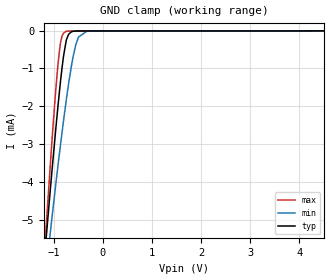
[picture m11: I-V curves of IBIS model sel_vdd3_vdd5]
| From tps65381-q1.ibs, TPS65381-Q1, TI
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|   sel_vdd3_vdd5 Model
[Model]   sel_vdd3_vdd5
Model_type   Input
Vinl = 0.99
Vinh = 2.31
|   typ   min   max
|   (nom PVT)   (fast PVT)   (slow PVT)
C_comp   3.884e-13   3.208e-13   3.942e-13
[Model spec]
|subparameter
Vinl   0.99   0.951   1.029
Vinh   2.31   2.219   2.401
| Where nom  PVT is Nominal Process, 3.3V, 27C
|   Fast PVT is Strong Process,  3.43V, -40C
|   Slow PVT is Weak Process,   3.17V, 150C
[Voltage Range]   3.3   3.17   3.43
|Junction Temperature
[Temperature Range]   27   150   -40
[Power Clamp Reference]   3.3   3.17   3.43
[GND Clamp Reference]   0   0   0
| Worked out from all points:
|   GND clamp passes 1 mA (typ) near -0.83 V on its own axis
[GND Clamp]
|   Voltage   I(typ)   I(min)   I(max)
-3.3V     -43.47mA   -34.59mA   -53.63mA
-1.187V   -5.949mA   -6.718mA   -5.768mA
-1.052V   -3.922mA   -5.116mA   -3.177mA
-910.8mV  -1.931mA   -3.517mA   -823.6uA
-871.6mV  -1.432mA   -3.095mA   -387.1uA
-833.8mV  -993.6uA   -2.701mA   -149.2uA
-749.1mV  -276.7uA   -1.862mA   -21.85uA
-646.8mV  -36.09uA   -972.7uA   -10.33uA
-554.8mV  -11.92uA   -381.6uA   -10.02uA
-497.7mV  -10.25uA   -171.8uA   -10uA
-330mV    -10uA      -18.55uA   -10uA
6.6V      0A         0A         0A
[POWER Clamp]
|   Voltage   I(typ)   I(min)   I(max)
-3.3V     0A         0A         0A
0V        0A         0A         0A
6.6V      0A         0A         0A
